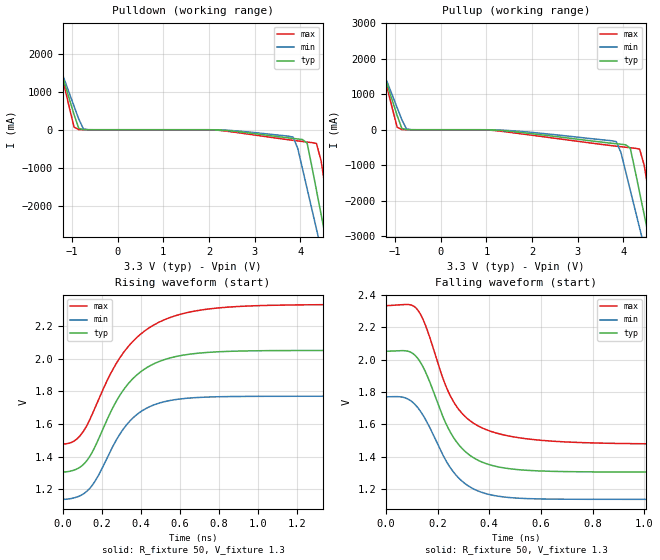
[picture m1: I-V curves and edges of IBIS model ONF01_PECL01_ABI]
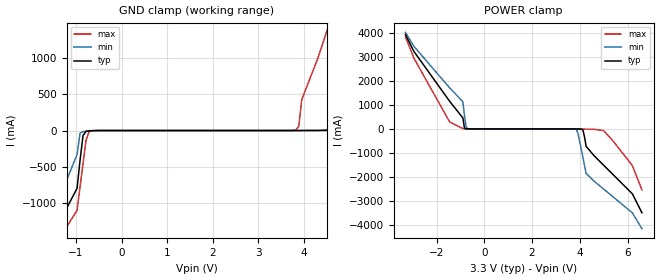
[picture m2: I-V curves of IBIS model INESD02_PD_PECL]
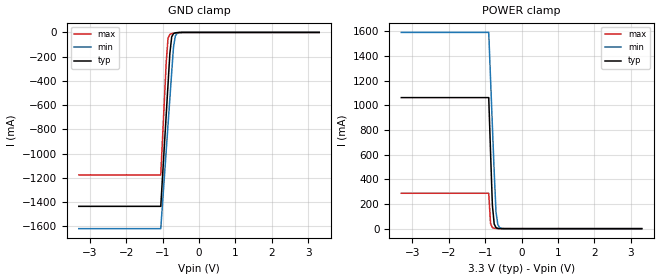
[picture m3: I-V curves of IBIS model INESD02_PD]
|   This file is an IBIS representation of the   |
|   Integrated Device Technology , Inc.   |
|   ICS9DB306   |
|   PCI Express Jitter Attenuator   |
[IBIS Ver]   4.1
[File name]   9db306_3v3.ibs
[File Rev]   1.0
[Date]   19 Oct 2009 | Last modified
|   Dec 03 2003 | Generated
[Source]   Originated at Integrated Device Technology, Inc.
[Disclaimer]
IDT hereby grants the user of this IBIS model a non-exclusive,
nontransferable license to use this IBIS model under the following terms.
Before using this IBIS model, the user should read this license.
If the user does not accept these terms,  the IBIS model should be
returned to IDT within 30 days.
   The user is granted this license only to use the IBIS model and
is not granted rights to sell, load, rent, lease or license the IBIS
model in whole or in part, or in modified form to anyone other than
user. User may modify the IBIS model to suit its specific
applications but rights to derivative works and such modifications
shall belong to IDT.
   This IBIS model is provided on an "AS IS" basis and IDT makes
absolutely no warranty with respect to the information contained
herein. IDT DISCLAIMS AND CUSTOMER WAIVES ALL WARRANTIES, EXPRESS
OR IMPLIED, INCLUDING WARRANTIES OF MERCHANTABILITY OR FITNESS FOR
A PARTICULAR PURPOSE. The entire risk as to quality and performance
is with the Customer. ACCORDINGLY, IN NO EVENT SHALL THE COMPANY BE
LIABLE FOR ANY DAMAGES, WHETHER IN CONTRACT OR TORT,INCLUDING ANY
LOST PROFITS OR OTHER INCIDENTAL, CONSEQUENTIAL, EXEMPLARY, OR
PUNITIVE DAMAGES ARISING OUT OF THE USE OR APPLICATION OF THE IBIS
model provided in this package. Further, IDT reserves the right to
make changes without notice to any product herein to improve
reliability, function, or design. IDT does not convey any license
under patent rights or any other intellectual property rights,
including those of third parties.
   IDT is not obligated to provide maintenance or support
for the licensed IBIS model.
[Copyright]   Copyright 2004 by Integrated Device Technology , Inc.
[Component]   ICS9DB306L
[Manufacturer] Integrated Device Technology, Inc.
[Package]
|TSSOP 28 Pin
|   typ   min   max
R_pkg   60.65m   52.4m   68.9m
L_pkg   1.989nH   1.431nH   2.547nH
C_pkg   0.314pF   0.254pF   0.374pF
[Pin]  signal_name   model_name   R_pin   L_pin   C_pin
1   VEE   GND   68.9m   2.547n   0.374p
2   PCIEXT1  ONF01_PECL01_ABI   66.2m   2.360n   0.254p
3   PCIEXC1  ONF01_PECL01_ABI   63.4m   2.174n   0.334p
4   PCIEXT2  ONF01_PECL01_ABI   60.6m   1.988n   0.314p
5   PCIEXC2  ONF01_PECL01_ABI   57.9m   1.802n   0.294p
6   VCC   POWER   55.1m   1.616n   0.274p
7   nOE0   INESD02_PD_PECL   52.4m   1.431n   0.254p
8   nOE1   INESD02_PD_PECL   52.4m   1.431n   0.254p
9   VCC   POWER   55.1m   1.616n   0.274p
10   PCIEXC3  ONF01_PECL01_ABI   57.9m   1.802n   0.294p
11   PCIEXT3  ONF01_PECL01_ABI   60.6m   1.988n   0.314p
12   PCIEXC4  ONF01_PECL01_ABI   63.4m   2.174n   0.334p
13   PCIEXT4  ONF01_PECL01_ABI   66.2m   2.360n   0.254p
14   VEE   GND   68.9m   2.547n   0.374p
15   VCC   POWER   68.9m   2.547n   0.374p
16   PCIEXC5  ONF01_PECL01_ABI   66.2m   2.360n   0.254p
17   PCIEXT5  ONF01_PECL01_ABI   63.4m   2.174n   0.334p
18   FS1   INESD02_PD_PECL   60.6m   1.988n   0.314p
19   BYPASS   INESD02_PD   57.9m   1.802n   0.294p
20   VEE   GND   55.1m   1.616n   0.274p
21   VCCA   POWER   52.4m   1.431n   0.254p
22   PLL_BW   INESD02_PU_PECL   52.4m   1.431n   0.254p
23   CLK   INESD02_PD_PECL   55.1m   1.616n   0.274p
24   nCLK   INESD02_PMID_PEC   57.9m   1.802n   0.294p
25   FS0   INESD02_PU_PECL   60.6m   1.988n   0.314p
26   PCIEXT0  ONF01_PECL01_ABI   63.4m   2.174n   0.334p
27   PCIEXC0  ONF01_PECL01_ABI   66.2m   2.360n   0.254p
28   VCC   POWER   68.9m   2.547n   0.374p
[Diff Pin]  inv_pin  vdiff tdelay_typ tdelay_min  tdelay_max
2   3   NA   0   0   0
4   5   NA   0   0   0
11   10   NA   0   0   0
13   12   NA   0   0   0
17   16   NA   0   0   0
23   24   0.15   0   0   0
26   27   NA   0   0   0
[Component]   ICS9DB306F
[Manufacturer] Integrated Device Technology, Inc.
[Package]
|SSOP 28 Pin
|   typ   min   max
R_pkg   69.7m   57.8m   81.6m
L_pkg   2.906nH   2.168nH   3.644nH
C_pkg   0.376pF   0.242pF   0.511pF
[Pin]   signal_name   model_name   R_pin   L_pin   C_pin
1   VEE   GND   79.3m   2.922n   0.427p
2   PCIEXT1  ONF01_PECL01_ABI   75.1m   2.702n   0.395p
3   PCIEXC1  ONF01_PECL01_ABI   70.9m   2.482n   0.362p
4   PCIEXT2  ONF01_PECL01_ABI   66.7m   2.262n   0.329p
5   PCIEXC2  ONF01_PECL01_ABI   62.5m   2.041n   0.297p
6   VCC   POWER   58.3m   1.821n   0.264p
7   nOE0   INESD02_PD_PECL   54.1m   1.601n   0.232p
8   nOE1   INESD02_PD_PECL   54.1m   1.601n   0.232p
9   VCC   POWER   58.3m   1.821n   0.264p
10   PCIEXC3  ONF01_PECL01_ABI   62.5m   2.041n   0.297p
11   PCIEXT3  ONF01_PECL01_ABI   66.7m   2.262n   0.329p
12   PCIEXC4  ONF01_PECL01_ABI   70.9m   2.482n   0.362p
13   PCIEXT4  ONF01_PECL01_ABI   75.1m   2.702n   0.395p
14   VEE   GND   79.3m   2.922n   0.427p
15   VCC   POWER   79.3m   2.922n   0.427p
16   PCIEXC5  ONF01_PECL01_ABI   75.1m   2.702n   0.395p
17   PCIEXT5  ONF01_PECL01_ABI   70.9m   2.482n   0.362p
18   FS1   INESD02_PD_PECL   66.7m   2.262n   0.329p
19   BYPASS   INESD02_PD   62.5m   2.041n   0.297p
20   VEE   GND   58.3m   1.821n   0.264p
21   VCCA   POWER   54.1m   1.601n   0.232p
22   PLL_BW   INESD02_PU_PECL   54.1m   1.601n   0.232p
23   CLK   INESD02_PD_PECL   58.3m   1.821n   0.264p
24   nCLK   INESD02_PMID_PEC   62.5m   2.041n   0.297p
25   FS0   INESD02_PU_PECL   66.7m   2.262n   0.329p
26   PCIEXT0  ONF01_PECL01_ABI   70.9m   2.482n   0.362p
27   PCIEXC0  ONF01_PECL01_ABI   75.1m   2.702n   0.395p
28   VCC   POWER   79.3m   2.922n   0.427p
[Diff Pin]  inv_pin  vdiff tdelay_typ tdelay_min  tdelay_max
2   3   NA   0   0   0
4   5   NA   0   0   0
11   10   NA   0   0   0
13   12   NA   0   0   0
17   16   NA   0   0   0
23   24   0.15   0   0   0
26   27   NA   0   0   0
| Models and submodels in the file (5): ONF01_PECL01_ABI (Output_ECL), INESD02_PD_PECL (Input), INESD02_PD (Input), INESD02_PU_PECL (Input), INESD02_PMID_PEC (Input)
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[Model]   ONF01_PECL01_ABI
Model_type  Output_ECL
Polarity   Non-Inverting
Vmeas = 1.63
Rref = 50
Cref = 0
Vref = 1.3
|Variable  typ   min   max
C_comp   2p   1.5p   2.5p
[Voltage Range]   3.3   3.135   3.465
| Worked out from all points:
|   rising waveform, R_fixture 50, V_fixture 1.3: 20-80 % time 218ps typ, 193ps min, 263ps max; typ from 1.31 V to 2.05 V
|   falling waveform, R_fixture 50, V_fixture 1.3: 20-80 % time 134ps typ, 136ps min, 142ps max; typ from 2.05 V to 1.31 V
| Open source, no load
|  Voltage   I(typ)   I(min)   I(max)
[Pulldown]
-3.3V     9.786A     8.425A     12.06A
-1.667V   3.247A     2.986A     3.704A
-1.463V   2.432A     2.308A     2.661A
-952.6mV  398mA      618.5mA    68.87mA
-850.5mV  36.63mA    281.6mA    4.032mA
3.844V    -229.1mA   -195.7mA   -279.4mA
4.151V    -352.7mA   -1.559A    -324.9mA
4.355V    -1.599A    -2.62A     -360.9mA
4.559V    -2.871A    -3.681A    -1.635A
4.661V    -3.508A    -4.211A    -2.446A
4.763V    -4.144A    -4.742A    -3.257A
6.6V      -15.69A    -14.35A    -17.99A
[Pullup]
-3.3V     9.786A     8.425A     12.06A
-1.565V   2.839A     2.647A     3.182A
-952.6mV  398mA      618.5mA    68.87mA
-850.5mV  36.63mA    281.6mA    4.032mA
-646.4mV  229.3uA    964.8uA    177.5uA
3.844V    -394.4mA   -337mA     -463.1mA
4.151V    -517.8mA   -1.701A    -507.4mA
4.355V    -1.764A    -2.763A    -542.7mA
4.559V    -3.036A    -3.825A    -1.816A
4.661V    -3.672A    -4.355A    -2.626A
4.763V    -4.308A    -4.886A    -3.437A
6.6V      -15.79A    -14.46A    -18.06A
[Ramp]
|   typ   min   max
dV/dt_r   0.596/0.354n   0.506/0.311n   0.684/0.427n
dV/dt_f   0.599/0.219n   0.507/0.219n   0.690/0.252n
R_load =   50.0000
[Rising Waveform]
R_fixture = 50
V_fixture = 1.3   | VCC_typ - 2V
V_fixture_max = 1.465   | VCC_max - 2V
V_fixture_min = 1.135   | VCC_min - 2V
C_fixture = 0.0p
| Time   typ   min   max
0s        1.306V     1.138V     1.478V
67.2ps    1.321V     1.15V      1.503V
126ps     1.379V     1.19V      1.597V
176.4ps   1.489V     1.271V     1.731V
247.8ps   1.679V     1.442V     1.915V
338.1ps   1.85V      1.61V      2.079V
430.5ps   1.946V     1.698V     2.18V
554.4ps   2.007V     1.745V     2.255V
936.6ps   2.049V     1.77V      2.324V
1.999ns   2.052V     1.771V     2.333V
[Falling Waveform]
R_fixture = 50
V_fixture = 1.3   | VCC_typ - 2V
V_fixture_max = 1.465   | VCC_max - 2V
V_fixture_min = 1.135   | VCC_min - 2V
C_fixture = 0.0p
| Time   typ   min   max
0s        2.052V     1.771V     2.334V
73.5ps    2.055V     1.765V     2.34V
119.7ps   2.015V     1.711V     2.314V
151.2ps   1.932V     1.637V     2.221V
224.7ps   1.633V     1.399V     1.868V
268.8ps   1.503V     1.293V     1.723V
336ps     1.398V     1.205V     1.611V
434.7ps   1.338V     1.157V     1.544V
806.4ps   1.307V     1.138V     1.486V
1.999ns   1.306V     1.138V     1.478V
[Model]   INESD02_PD_PECL
Model_type  Input
Polarity   Non-Inverting
Vinl = 0.8V
Vinh = 2.0V
|   typ   min   max
C_comp   2pF   1.5pF   2.5pF
|   typ   min   max
[Voltage range]  3.3V   3.15V   3.45V
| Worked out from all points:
|   GND clamp passes 1 mA (typ) near -0.59 V on its own axis
|   POWER clamp passes 1 mA (typ) near -0.70 V on its own axis
[GND_clamp]
-3.3V     -3.894A    -4.294A    -3.674A
-1.6V     -1.569A    -1.322A    -1.74A
-974.8mV  -794.1mA   -331.5mA   -1.096A
-843.4mV  -68.33mA   -15.34mA   -452.9mA
-646.5mV  -1.912mA   -4.151mA   -2.665mA
3.818V    89.38uA    70.49uA    7.198mA
3.95V     342.2uA    75.94uA    423.8mA
4.6V      7.437mA    165.5uA    1.553A
4.9V      78.32mA    440.9uA    2.118A
5.5V      1.293A     2.769mA    3.249A
6.25V     2.651A     112.4mA    4.38A
6.6V      3.331A     896.1mA    4.946A
[POWER_clamp]
-3.3V     3.923A     4.017A     3.838A
-2.95V    3.23A      3.44A      2.951A
-1.45V    1.149A     1.709A     289.6mA
-896.9mV  456.5mA    1.133A     15.4mA
-762.9mV  4.223mA    91.07mA    1.486mA
-695.9mV  792.2uA    10.73mA    555.6uA
3.861V    -556.7uA   -26.14mA   -39.45uA
4.129V    -41.85mA   -1.19A     -4.904mA
4.263V    -724.2mA   -1.847A    -12.04mA
5V        -1.514A    -2.505A    -71.38mA
6.2V      -2.701A    -3.492A    -1.525A
6.6V      -3.492A    -4.151A    -2.536A
[Model]   INESD02_PD
Model_type   Input
Polarity   Non-Inverting
Vinl = 0.80V
Vinh = 2.0V
|   typ   min   max
C_comp   2pF   1.5pF   2.5pF
|   typ   min   max
[Voltage range]  3.3V   3.15V   3.45V
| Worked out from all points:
|   GND clamp passes 1 mA (typ) near -0.56 V on its own axis
|   POWER clamp passes 1 mA (typ) near -0.61 V on its own axis
[GND_clamp]
|Voltage   I(typ)   I(min)   I(max)
-3.3V     -1.436A    -1.62A     -1.176A
-1.05V    -1.436A    -1.62A     -1.176A
-900mV    -678.5mA   -975.1mA   -244mA
-850mV    -426.1mA   -760.1mA   -46.85mA
-800mV    -173.9mA   -545.4mA   -16.11mA
-750mV    -36.96mA   -330.7mA   -9.916mA
-700mV    -9.696mA   -120.2mA   -7.056mA
-650mV    -3.545mA   -29.7mA    -4.857mA
-600mV    -1.629mA   -7.52mA    -3.049mA
-400mV    -52.81uA   -52.52uA   -108.7uA
3.3V      71.13uA    77.43uA    62.11uA
[POWER_clamp]
|Voltage   I(typ)   I(min)   I(max)
-3.3V     1.063A     1.593A     287.3mA
-900mV    1.063A     1.593A     287.3mA
-850mV    620.5mA    1.215A     41.84mA
-800mV    191.6mA    837.5mA    8.757mA
-750mV    37.76mA    460.2mA    3.328mA
-700mV    8.104mA    133.8mA    1.728mA
-650mV    2.076mA    32.66mA    905.3uA
-600mV    678.1uA    8.083mA    443.8uA
-450mV    104.2uA    213.3uA    89.09uA
3.3V      -3.041nA   -3.986uA   0A
